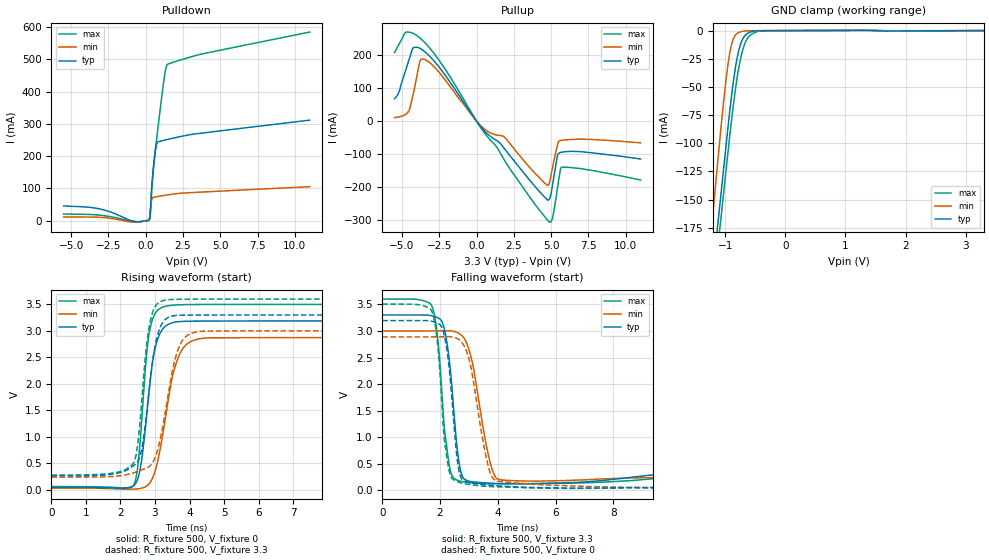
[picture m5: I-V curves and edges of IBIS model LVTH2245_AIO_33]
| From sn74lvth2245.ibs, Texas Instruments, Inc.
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[Model]   LVTH2245_AIO_33
Model_type  I/O
Vinl = 0.8
Vinh = 2.34
Enable   Active-Low
Vref =   0
Rref =   500
Cref =   50p
Vmeas =   1.5
| variable   typ   min   max
C_comp   6.48pF   5.16pF   8.61pF
| C_pullup   5.47pF   0.62pF   8.15pF
| C_pulldown   9.98pF   1.70pF   31.46pF
| C_tri-state   6.48pF   5.16pF   8.61pF
[Temperature Range]   40   -40   100
| Ambient temperature   25   -40   85
[Voltage range]   3.3   3   3.6
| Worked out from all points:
|   slope of the pulldown table from 0 to 0.495 V, typ, clamps not added: 3.18 ohm
|   slope of the pullup table from 0 to 0.495 V, typ, clamps not added: 17.9 ohm
|   GND clamp passes 1 mA (typ) near -0.56 V on its own axis
|   rising waveform, R_fixture 500, V_fixture 0: 20-80 % time 329ps typ, 476ps min, 251ps max; typ from 0.04 V to 3.19 V
|   falling waveform, R_fixture 500, V_fixture 3.3: 20-80 % time 314ps typ, 524ps min, 297ps max; typ from 3.3 V to 0.257 V
|   rising waveform, R_fixture 500, V_fixture 3.3: 20-80 % time 354ps typ, 483ps min, 282ps max; typ from 0.26 V to 3.3 V
|   falling waveform, R_fixture 500, V_fixture 0: 20-80 % time 317ps typ, 538ps min, 303ps max; typ from 3.2 V to 0.04 V
[GND Clamp]
| LVTH2245_AIO_33
|   Voltage   I(typ)   I(min)   I(max)
-5.5V     -2.907A    -3.062A    -2.915A
-1.25V    -238.4mA   -189.8mA   -258.9mA
-1.18V    -202.2mA   -149.5mA   -222.6mA
-1.075V   -148.4mA   -89.72mA   -169.6mA
-975mV    -97.46mA   -39.38mA   -119.6mA
-900mV    -61.04mA   -13.9mA    -82.84mA
-825mV    -31.8mA    -3.71mA    -50.88mA
-775mV    -18.18mA   -1.733mA   -33.88mA
-700mV    -6.661mA   -663.2uA   -15.71mA
-625mV    -2.392mA   -221.1uA   -6.629mA
-300mV    -69.5uA    -61.23uA   -87.84uA
3.3V      36.14pA    29.21pA    -1.136uA
[Pulldown]
| LVTH2245_AIO_33
|   Voltage   I(typ)   I(min)   I(max)
-5.5V     45.68mA    11.37mA    20.79mA
-3.04V    35.93mA    10.33mA    16.91mA
-690mV    -3.193mA   -4.66mA    -2.388mA
245mV     3.455mA    8.012mA    3.33mA
315mV     33.13mA    35.96mA    22.68mA
425mV     118.9mA    68.08mA    110mA
580mV     192.7mA    73.08mA    190.3mA
710mV     233.6mA    74.13mA    244.7mA
1.245V    249.3mA    78.27mA    443.5mA
1.365V    250.6mA    79.15mA    474.6mA
1.47V     251.8mA    79.9mA     484.6mA
11V       311.5mA    105.3mA    584.3mA
[Pullup]
| LVTH2245_AIO_33
|   Voltage   I(typ)   I(min)   I(max)
-5.5V     67.92mA    10.82mA    207.4mA
-4.615V   173.6mA    26.44mA    269.3mA
-4.28V    220.1mA    75.69mA    266.1mA
-3.79V    220mA      182.9mA    251.2mA
-3.465V   209.8mA    186.5mA    237.2mA
270mV     -15.96mA   -13.16mA   -19.22mA
1.855V    -82.19mA   -47.41mA   -116.7mA
4.89V     -235.3mA   -184.7mA   -304.8mA
5.11V     -188.9mA   -136.1mA   -288.5mA
5.435V    -102.2mA   -70.96mA   -199.1mA
5.69V     -93.81mA   -57.8mA    -139.6mA
11V       -114.3mA   -65.47mA   -177.8mA
[Ramp]
| LVTH2245_AIO_33
| variable   typ   min   max
dV/dt_r   1.90/3.42E-10   1.72/4.85E-10   2.08/2.56E-10
dV/dt_f   1.90/3.33E-10   1.70/5.44E-10   2.09/3.22E-10
R_load = 500
[Rising Waveform]
| LVTH2245_AIO_33
R_fixture =   500
C_fixture =   0
L_fixture =   0
V_fixture =   0
V_fixture_min = 0
V_fixture_max = 0
|   Time   V(typ)   V(min)   V(max)
0s        40.37mV    24.11mV    55.61mV
2.375ns   69.73mV    7.165mV    71.08mV
2.595ns   478.7mV    24.17mV    1.116V
2.74ns    1.28V      57.6mV     2.432V
2.855ns   2.011V     128.1mV    3.035V
3.085ns   2.856V     557mV      3.393V
3.49ns    3.149V     2.089V     3.482V
3.885ns   3.18V      2.726V     3.495V
4.625ns   3.184V     2.868V     3.498V
50ns      3.188V     2.873V     3.5V
[Falling Waveform]
| LVTH2245_AIO_33
R_fixture =   500
C_fixture =   0
L_fixture =   0
V_fixture =   3.3
V_fixture_min = 3
V_fixture_max = 3.6
|   Time   V(typ)   V(min)   V(max)
0s        3.3V       3V         3.6V
1.705ns   3.287V     3.001V     3.482V
1.895ns   3.255V     3.001V     2.98V
2.06ns    3.185V     3.002V     1.87V
2.375ns   2.172V     3.001V     337.5mV
2.66ns    523.9mV    2.954V     181.2mV
2.95ns    182.7mV    2.733V     150.7mV
3.725ns   137.1mV    547.7mV    126.8mV
4.155ns   129.2mV    194.4mV    125.4mV
50ns      257mV      233.5mV    268.7mV
[Rising Waveform]
| LVTH2245_AIO_33
R_fixture =   500
C_fixture =   0
L_fixture =   0
V_fixture =   3.3
V_fixture_min = 3
V_fixture_max = 3.6
|   Time   V(typ)   V(min)   V(max)
0s        260.5mV    234.6mV    273.1mV
2.385ns   453.5mV    316.6mV    509.6mV
2.5ns     526.7mV    344.2mV    852.2mV
2.615ns   761.9mV    372.9mV    1.657V
2.855ns   2.019V     446.5mV    3.154V
3.07ns    2.905V     732.6mV    3.512V
3.38ns    3.251V     1.783V     3.588V
3.765ns   3.295V     2.787V     3.597V
4.45ns    3.298V     2.994V     3.599V
50ns      3.3V       3V         3.6V
[Falling Waveform]
| LVTH2245_AIO_33
R_fixture =   500
C_fixture =   0
L_fixture =   0
V_fixture =   0
V_fixture_min = 0
V_fixture_max = 0
|   Time   V(typ)   V(min)   V(max)
0s        3.196V     2.888V     3.505V
1.705ns   3.183V     2.888V     3.385V
1.89ns    3.152V     2.889V     2.878V
2.055ns   3.078V     2.89V      1.716V
2.31ns    2.338V     2.892V     383.3mV
2.655ns   372.8mV    2.836V     152.9mV
3.12ns    133.7mV    2.17V      102.5mV
3.76ns    95.97mV    301.8mV    73.32mV
4.685ns   64.78mV    137.1mV    55.88mV
50ns      40.13mV    24.04mV    55.6mV
